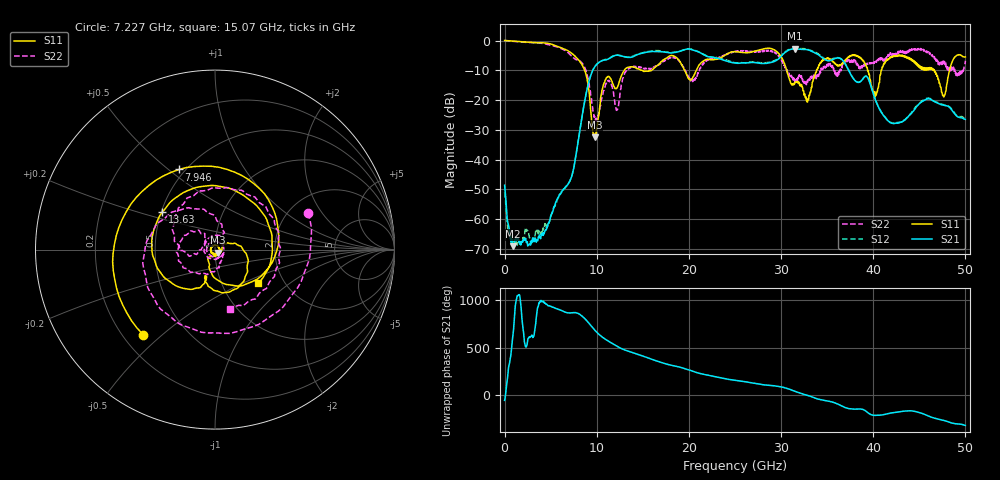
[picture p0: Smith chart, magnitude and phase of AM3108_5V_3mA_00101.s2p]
# Hz S DB R 50.0
!freq dBS11 angS11 dBS21 angS21 dBS12 angS12 dBS22 angS22
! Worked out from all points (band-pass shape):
!   1601 points, 10 MHz to 50 GHz, reference 50 ohm
!   highest |S21| = -2.79 dB at 31.53 GHz (marker M1); lowest = -69.0 dB at 947.3 MHz (marker M2)
!   |S21| within 3 dB of the highest: 11.49 GHz to 22.83 GHz (11.34 GHz wide, 66.1 % of centre); 29.86 GHz to 34.47 GHz (4.61 GHz wide, 14.3 % of centre)
!   lowest |S11| = -32.5 dB at 9.789 GHz (marker M3), VSWR 1.05, Z = 51.7 - j1.74 ohm
!   |S11| at or under -10 dB: 8.698 GHz to 12.99 GHz (4.289 GHz wide, 39.6 % of centre); 30.63 GHz to 33.85 GHz (3.219 GHz wide, 9.98 % of centre); 46.63 GHz to 48.28 GHz (1.653 GHz wide, 3.48 % of centre)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
!   |S22| runs from -27.5 to 0.0 dB; largest |S21 - S12| = 0.027
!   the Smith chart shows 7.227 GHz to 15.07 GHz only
!   S11 on the Smith chart (normalised r, x): 7.227 GHz: 0.28, -0.43; 7.946 GHz: 0.46, +0.54; 13.63 GHz: 0.51, +0.24; 15.07 GHz: 1.48, -0.61
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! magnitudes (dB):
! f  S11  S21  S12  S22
! 10 MHz  0.0  -48.6  -50.9  0.0
! 947.3 MHz  -0.2  -69.0  -67.5  -0.3
! 4.072 GHz  -0.7  -65.1  -64.4  -1.0
! 7.227 GHz  -4.1  -46.1  -46.2  -5.1
! 7.946 GHz  -6.2  -34.6  -34.5  -6.7
! 8.352 GHz  -7.8  -26.7  -26.6  -7.3
! 9.789 GHz  -32.5  -8.8  -8.8  -25.6
! 10.95 GHz  -13.1  -6.5  -6.4  -14.9
! 12.23 GHz  -15.8  -4.9  -4.8  -23.3
! 13.63 GHz  -8.9  -5.7  -5.5  -9.1
! 15.07 GHz  -10.4  -4.1  -4.0  -9.4
! 16.69 GHz  -8.1  -3.7  -3.4  -8.3
! 20.41 GHz  -12.4  -3.2  -3.0  -13.8
! 25 GHz  -3.7  -7.5  -7.4  -3.8
! 29.16 GHz  -2.9  -7.2  -6.9  -3.6
! 31.53 GHz  -14.1  -2.8  -2.7  -13.9
! 33.35 GHz  -15.6  -3.6  -3.4  -12.7
! 38 GHz  -4.8  -13.4  -13.4  -6.6
! 40.22 GHz  -18.8  -19.8  -19.7  -7.6
! 41.69 GHz  -6.1  -27.2  -27.0  -5.2
! 47.66 GHz  -18.9  -21.8  -21.6  -7.7
! 50 GHz  -5.5  -26.5  -26.3  -6.8
